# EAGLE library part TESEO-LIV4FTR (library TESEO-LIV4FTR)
Tiny dual-band GNSS low power and measurement engine modules Source: Datasheet
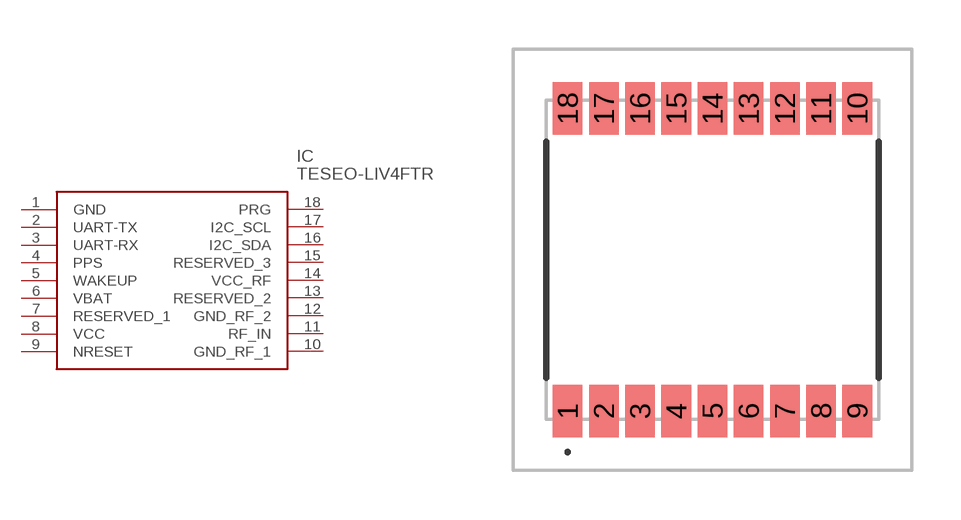
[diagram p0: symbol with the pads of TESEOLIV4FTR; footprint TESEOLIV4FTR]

Designator prefix IC

## TESEO-LIV4FTR (Arrow_Part_Number: TESEO-LIV4FTR; Arrow_Price-Stock: https://www.arrow.com/en/products/teseo-liv4ftr/stmicroelectronics?utm_currency=USD&region=nac; Description: Tiny dual-band GNSS low power and measurement engine modules; Height: 2.3mm; Manufacturer_Name: STMicroelectronics; Manufacturer_Part_Number: TESEO-LIV4FTR; Mouser_Part_Number: 511-TESEO-LIV4FTR; Mouser_Price-Stock: https://www.mouser.co.uk/ProductDetail/STMicroelectronics/TESEO-LIV4FTR?qs=By6Nw2ByBD3%252BjjBvGBu5LQ%3D%3D)  [TESEOLIV4FTR]
1  GND
2  UART-TX
3  UART-RX
4  PPS
5  WAKEUP
6  VBAT
7  RESERVED_1
8  VCC
9  NRESET
10  GND_RF_1
11  RF_IN
12  GND_RF_2
13  RESERVED_2
14  VCC_RF
15  RESERVED_3
16  I2C_SDA
17  I2C_SCL
18  PRG

## Footprint TESEOLIV4FTR (pad centres in mm)
TESEO-LIV4FTR-1
smd 0.9 x 1.6: 1 -4.4,-4.6; 2 -3.3,-4.6; 3 -2.2,-4.6; 4 -1.1,-4.6; 5 0,-4.6; 6 1.1,-4.6; 7 2.2,-4.6; 8 3.3,-4.6; 9 4.4,-4.6; 10 4.4,4.6; 11 3.3,4.6; 12 2.2,4.6; 13 1.1,4.6; 14 0,4.6; 15 -1.1,4.6; 16 -2.2,4.6; 17 -3.3,4.6; 18 -4.4,4.6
